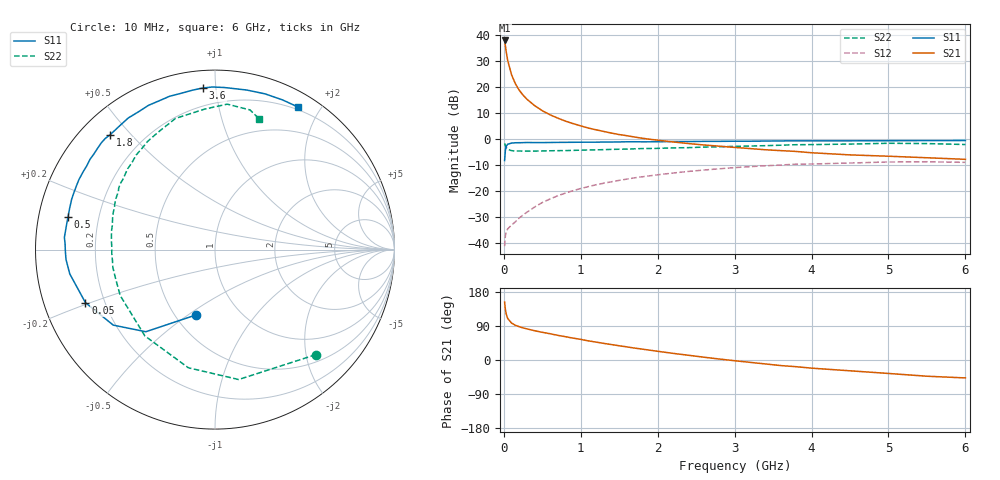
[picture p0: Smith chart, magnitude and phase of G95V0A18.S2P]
! SIEMENS Small Signal Semiconductors
! BFG235
! Si NPN RF Bipolar Junction Transistor in SOT223
! VCE = 5 V  IC = 180 mA
! Common Emitter S-Parameters:  July  1994
# GHz  S  MA  R  50
!  f  S11  S21  S12  S22
! GHz  MAG  ANG  MAG  ANG  MAG  ANG  MAG  ANG
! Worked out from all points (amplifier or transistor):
!   40 points, 10 MHz to 6 GHz, reference 50 ohm
!   highest |S21| = 37.8 dB at 10 MHz (marker M1)
!   |S21| within 3 dB of that: start of sweep to 24.57 MHz
!   unconditionally stable (mu >= 1): 443 MHz to 1.5 GHz
!   at 200 MHz: K = 0.82, MSG = 24.6 dB, |S12| = -30.6 dB
!   at 1.5 GHz: K = 1.00, MAG = 8.8 dB, |S12| = -16.1 dB
!   at 6 GHz: K = 0.90, MSG = 0.6 dB, |S12| = -9.1 dB
!   S11 on the Smith chart (normalised r, x): 10 MHz: 0.63, -0.54; 50 MHz: 0.13, -0.19; 500 MHz: 0.09, +0.11; 1.8 GHz: 0.09, +0.44; 3.6 GHz: 0.09, +0.92; 6 GHz: 0.17, +1.73
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0.01  0.3782 -106.0  77.53 152.8  0.0085 61.6  0.8112 -46.2
0.02  0.5982 -130.1  61.26 133.9  0.0134 49.0  0.7357 -79.7
0.03  0.7059 -143.4  48.16 122.0  0.016 41.3  0.6749 -102.7
0.05  0.7799 -157.7  32.13 109.5  0.0183 34.7  0.6196 -129.1
0.1  0.8204 -170.5  16.98 97.5  0.0217 39.2  0.5869 -154.2
0.15  0.8321 -176.3  11.4 91.6  0.025 45.7  0.5768 -164.7
0.2  0.8338 -179.5  8.529 87.9  0.0296 50.3  0.5776 -170.2
0.25  0.8361 177.6  6.874 84.7  0.0338 54.0  0.5744 -174.0
0.3  0.8419 175.4  5.736 82.2  0.0383 57.1  0.5755 -177.3
0.4  0.8386 171.0  4.314 77.3  0.0482 59.7  0.5753 178.5
0.5  0.8391 167.4  3.445 73.0  0.0589 61.2  0.5794 175.0
0.6  0.8416 164.4  2.878 69.4  0.0688 61.2  0.5829 171.8
0.7  0.8463 160.8  2.483 65.1  0.0793 61.1  0.5864 169.1
0.9  0.8498 155.3  1.945 57.8  0.0995 58.7  0.5934 164.3
1.1  0.8532 149.1  1.595 50.4  0.1193 55.9  0.6041 159.5
1.8  0.8669 132.3  1.016 28.7  0.1841 43.8  0.643 145.2
2.2  0.8782 123.4  0.863 17.5  0.2173 36.2  0.6629 137.3
3.2  0.891 102.3  0.643 -6.2  0.2884 16.8  0.7185 118.5
3.6  0.903 94.3  0.587 -14.7  0.3106 8.3  0.746 110.3
4.5  0.9065 78.7  0.486 -28.5  0.339 -7.8  0.7849 94.2
5.5  0.915 65.7  0.428 -42.8  0.3588 -25.9  0.8022 75.9
6  0.9191 59.8  0.399 -47.3  0.3488 -32.6  0.7693 71.4
